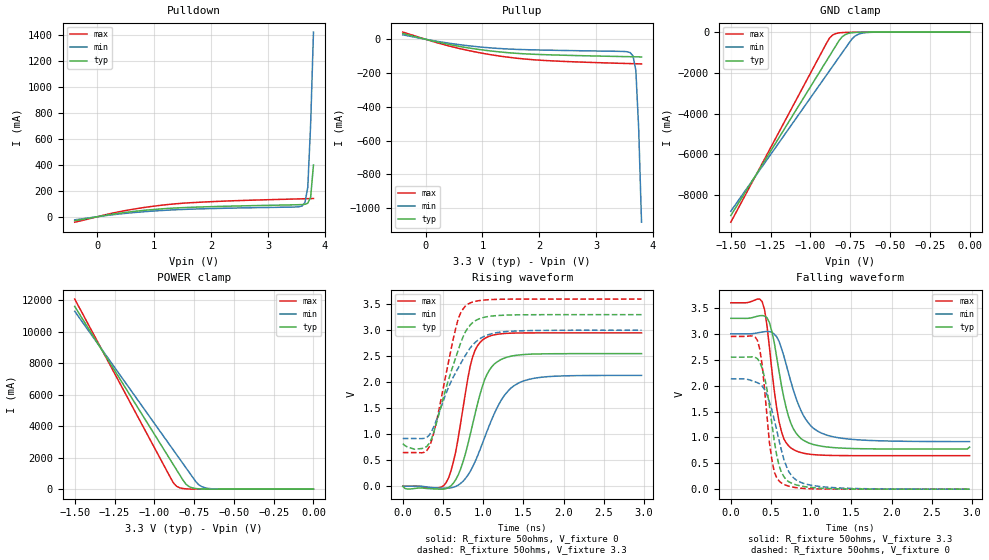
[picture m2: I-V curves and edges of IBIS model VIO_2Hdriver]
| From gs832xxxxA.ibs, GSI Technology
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|  signals   DQA1-DQA9, DQB1-DQB9, DQC1-DQC9, DQD1-DQD9
[Model]   VIO_2Hdriver
Model_type   I/O
Polarity   Non-Inverting
Vinl  =   0.8v
Vinh  =   2.0v
Vmeas =   1.5v
Cref  =   0pF
Rref  =   50
Vref  =   1.5v
|  variable   typ   min   max
C_comp   3.0pF   2.5pF   3.5pF
|  variable   typ   min   max
[Temperature Range]   50   0   100
|  variable   typ   min   max
[Voltage Range]   3.3   3.0   3.6
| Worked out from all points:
|   slope of the pulldown table from 0 to 0.495 V, typ, clamps not added: 14.9 ohm
|   slope of the pullup table from 0 to 0.495 V, typ, clamps not added: 13.7 ohm
|   GND clamp passes 1 mA (typ) near -0.58 V on its own axis
|   POWER clamp passes 1 mA (typ) near -0.61 V on its own axis
|   rising waveform, R_fixture 50ohms, V_fixture 0: 20-80 % time 259ps typ, 360ps min, 200ps max; typ from -0.004 V to 2.55 V
|   rising waveform, R_fixture 50ohms, V_fixture 3.3: 20-80 % time 295ps typ, 372ps min, 237ps max; typ from 0.816 V to 3.3 V
|   falling waveform, R_fixture 50ohms, V_fixture 3.3: 20-80 % time 195ps typ, 281ps min, 150ps max; typ from 3.3 V to 0.812 V
|   falling waveform, R_fixture 50ohms, V_fixture 0: 20-80 % time 157ps typ, 220ps min, 117ps max; typ from 2.55 V to 0 V
[Pulldown]
| voltage   typ   min   max
-400mV    -30.72mA   -24mA      -42.23mA
450mV     30.66mA    23.82mA    43.83mA
1.25V     63.98mA    50.77mA    94.11mA
2.15V     79.28mA    64.15mA    118.5mA
3.45V     91.34mA    74.34mA    136mA
3.6V      93.44mA    82.75mA    137.7mA
3.65V     95.64mA    109mA      138.3mA
3.7V      104.2mA    227.3mA    138.9mA
3.75V     149.3mA    708.4mA    139.4mA
3.8V      398.5mA    1.421A     140mA
[Pullup]
| voltage (VDDQ-Vout) typ   min   max
-400mV    33.83mA    26.51mA    42.45mA
500mV     -36.45mA   -27.62mA   -47.09mA
900mV     -58.59mA   -43.73mA   -76.65mA
1.35V     -76.47mA   -55.83mA   -101.8mA
2.1V      -91.36mA   -64.35mA   -125.9mA
3.45V     -102.4mA   -71.92mA   -142.8mA
3.6V      -103.4mA   -79.01mA   -144.2mA
3.65V     -103.7mA   -98.71mA   -144.7mA
3.7V      -104.1mA   -183.9mA   -145.1mA
3.75V     -104.4mA   -528.8mA   -145.6mA
3.8V      -104.9mA   -1.084A    -146mA
[GND Clamp]
| voltage   typ   min   max
-1.5V     -9.007A    -8.796A    -9.334A
-900mV    -1.431A    -2.122A    -562.9mA
-880mV    -1.176A    -1.9A      -292.9mA
-860mV    -920.8mA   -1.678A    -142.5mA
-820mV    -419.7mA   -1.233A    -38.58mA
-800mV    -224.7mA   -1.011A    -23.51mA
-780mV    -119.5mA   -788.8mA   -16.2mA
-740mV    -33.04mA   -348.7mA   -9.876mA
-720mV    -18.57mA   -198.2mA   -8.142mA
-680mV    -6.87mA    -61.92mA   -5.539mA
-580mV    -1.002mA   -3.885mA   -1.438mA
0V        -616.9pA   -1.102nA   -625.8pA
[POWER Clamp]
| voltage (VDDQ-Vout)  typ   min   max
-1.5V     11.62A     11.31A     12.09A
-900mV    1.877A     2.768A     763.5mA
-880mV    1.553A     2.483A     398.4mA
-860mV    1.228A     2.198A     183.4mA
-840mV    903.6mA    1.913A     83.63mA
-800mV    304.2mA    1.344A     19.43mA
-780mV    154.7mA    1.059A     10.68mA
-740mV    39.51mA    489.9mA    4.639mA
-720mV    20.32mA    274.5mA    3.532mA
-680mV    5.894mA    82.85mA    2.298mA
-580mV    568.7uA    4.201mA    684.1uA
0V        917.2pA    2.697nA    666.9pA
[Ramp]
| voltage   typ   min   max
dV/dt_r   1.08/117p   0.93/150p   1.27/94p
dV/dt_f   1.09/118p   0.92/150p   1.29/94p
R_load  =   50ohms
[Rising Waveform]
C_fixture =   0.0pf
R_fixture =   50ohms
V_fixture =   0
| Time   V(typ)   V(min)   V(max)
0s        -3.777mV   13.55nV    4.688nV
540ps     -46.65mV   -38.74mV   70.55mV
600ps     8.333mV    -31.39mV   295mV
690ps     217.8mV    21.76mV    932.2mV
810ps     807.6mV    211.8mV    2.08V
870ps     1.198V     375.4mV    2.49V
1.02ns    2.055V     942.6mV    2.843V
1.26ns    2.462V     1.738V     2.937V
1.5ns     2.532V     2.024V     2.948V
2.97ns    2.55V      2.132V     2.95V
[Rising Waveform]
C_fixture =   0.0pf
R_fixture =   50ohms
V_fixture =   3.3
V_fixture_min =   3.0
V_fixture_max =   3.6
| Time   V(typ)   V(min)   V(max)
0s        816.4mV    917.5mV    646.8mV
150ps     710.1mV    917.4mV    647mV
330ps     826.1mV    984.1mV    758.4mV
420ps     1.218V     1.276V     1.252V
570ps     2.049V     1.906V     2.398V
690ps     2.618V     2.276V     3.221V
810ps     3.044V     2.595V     3.502V
990ps     3.24V      2.865V     3.578V
1.23ns    3.287V     2.967V     3.597V
2.97ns    3.3V       3V         3.6V
[Falling Waveform]
C_fixture =   0.0pf
R_fixture =   50ohms
V_fixture =   3.3
V_fixture_min =   3.0
V_fixture_max =   3.6
| Time   V(typ)   V(min)   V(max)
0s        3.3V       3V         3.6V
390ps     3.354V     3.035V     3.621V
420ps     3.345V     3.042V     3.466V
480ps     3.22V      3.043V     2.749V
600ps     2.276V     2.855V     1.304V
660ps     1.767V     2.572V     969.5mV
750ps     1.261V     2.06V      793.6mV
930ps     922.1mV    1.354V     686.9mV
1.2ns     814.4mV    1.041V     653.4mV
2.97ns    811.7mV    918.5mV    646.9mV
[Falling Waveform]
C_fixture =   0.0pf
R_fixture =   50ohms
V_fixture =   0
| Time   V(typ)   V(min)   V(max)
0s        2.55V      2.13V      2.95V
330ps     2.522V     2.057V     2.879V
390ps     2.332V     1.99V      2.395V
480ps     1.611V     1.688V     907.3mV
510ps     1.274V     1.532V     579mV
570ps     661.9mV    1.148V     225.3mV
630ps     324.3mV    747.7mV    119.8mV
750ps     119.6mV    274mV      46.35mV
990ps     34.6mV     79mV       8.038mV
2.97ns    4.357uV    167.4uV    181.3nV
